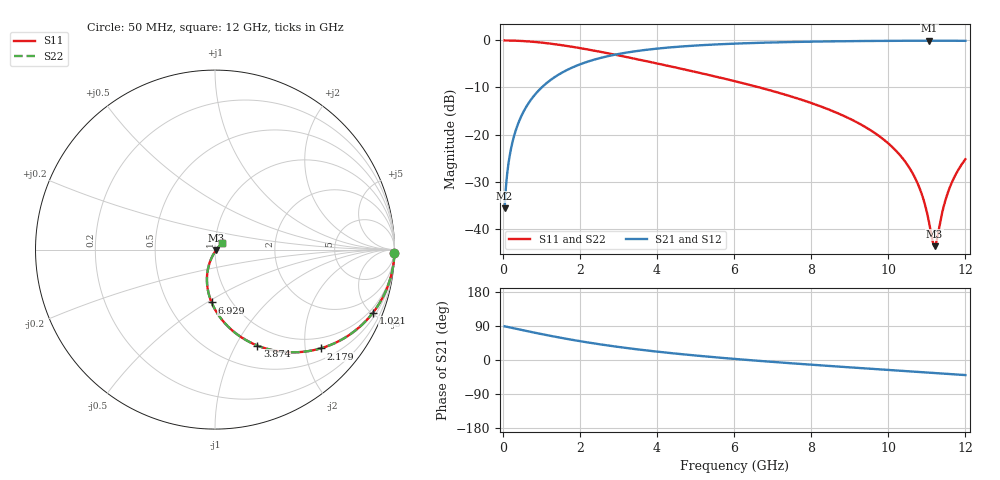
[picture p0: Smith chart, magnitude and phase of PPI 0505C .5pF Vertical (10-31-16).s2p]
# GHz S MA R 50
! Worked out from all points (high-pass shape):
!   1601 points, 50 MHz to 12 GHz, reference 50 ohm
!   highest |S21| = -0.06 dB at 11.07 GHz (marker M1); lowest = -35.7 dB at 50 MHz (marker M2)
!   |S21| within 3 dB of the highest: 2.89 GHz to end of sweep
!   lowest |S11| = -43.7 dB at 11.2 GHz (marker M3), VSWR 1.01, Z = 50.5 - j0.378 ohm
!   |S11| at or under -10 dB: 6.661 GHz to end of sweep
!   |S22| runs from -43.7 to 0.0 dB; largest |S21 - S12| = 0
!   S11 on the Smith chart (normalised r, x): 50 MHz: open; 1.021 GHz: 0.74, -5.08; 2.179 GHz: 0.74, -2.33; 3.874 GHz: 0.76, -1.23; 6.929 GHz: 0.81, -0.52; 12 GHz: 1.08, +0.08
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0.05  0.9999 -1.1  0.01641 88.9  0.01641 88.9  0.9999 -1.1
0.1844375  0.9982 -4.0  0.06042 85.9  0.06042 85.9  0.9982 -4.0
0.3562187  0.9932 -7.8  0.1162 82.2  0.1162 82.2  0.9932 -7.8
0.6325625  0.9789 -13.8  0.2036 76.2  0.2036 76.2  0.9789 -13.8
1.020938  0.9474 -21.8  0.3191 68.1  0.3191 68.1  0.9474 -21.8
2.044156  0.824 -40.9  0.5648 49.0  0.5648 49.0  0.824 -40.9
2.178594  0.8057 -43.1  0.5904 46.8  0.5904 46.8  0.8057 -43.1
3.874  0.5845 -66.2  0.8083 23.6  0.8083 23.6  0.5845 -66.2
4.038312  0.5654 -68.0  0.8217 21.7  0.8217 21.7  0.5654 -68.0
6.025  0.3686 -86.6  0.9253 2.7  0.9253 2.7  0.3686 -86.6
6.928719  0.2953 -93.6  0.9506 -4.5  0.9506 -4.5  0.2953 -93.6
8.019156  0.215 -101.2  0.9713 -12.5  0.9713 -12.5  0.215 -101.2
9.184281  0.1349 -108.4  0.9849 -20.7  0.9849 -20.7  0.1349 -108.4
10.01331  0.07961 -112.1  0.9904 -26.3  0.9904 -26.3  0.07961 -112.1
10.6855  0.03517 -110.7  0.9925 -30.9  0.9925 -30.9  0.03517 -110.7
10.90209  0.02111 -104.9  0.9928 -32.3  0.9928 -32.3  0.02111 -104.9
11.06641  0.01116 -88.3  0.9928 -33.4  0.9928 -33.4  0.01116 -88.3
11.20084  0.006499 -35.2  0.9928 -34.4  0.9928 -34.4  0.006499 -35.2
11.25313  0.007373 -7.0  0.9928 -34.7  0.9928 -34.7  0.007373 -7.0
11.42491  0.01642 30.3  0.9926 -35.9  0.9926 -35.9  0.01642 30.3
11.57428  0.02602 38.2  0.9923 -36.9  0.9923 -36.9  0.02602 38.2
12  0.05463 42.9  0.9908 -39.8  0.9908 -39.8  0.05463 42.9
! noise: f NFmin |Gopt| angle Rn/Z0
0.05  0.001875  0.9838  1.02  0.0264
1.372  0.005898  0.7838  8.43  0.005572
2.701  0.009101  0.7212  12.01  0.006401
4.031  0.01197  0.6864  15.59  0.007281
5.36  0.01469  0.664  19.18  0.008154
6.682  0.01735  0.6491  22.72  0.00904
8.012  0.02004  0.6396  26.23  0.009982
9.341  0.0228  0.6345  29.67  0.01101
10.67  0.02569  0.633  33.04  0.01215
12  0.02875  0.6348  36.34  0.01345
